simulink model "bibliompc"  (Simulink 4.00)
settings: Solver=ode45  StartTime=0.0  StopTime=10.0  RelTol=1e-3
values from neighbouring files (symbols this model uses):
  m = p    (= 10)    [scr.m]    (also in Smpc.m = mp(1:max(size(mp))-1); demo1dat.m = 4; demo2dat.m = 3; essai1dat.m = 4)
  model = [y(2:ly); 1; 1; .1]    [scr.m]    (also in Smpc.m = modelpd(:,1:nu); essai2dat.m = tfd2step(1.6,delt,1,g); mynlcmpc.m = modelpd(:,1:nu); mynlcmpc2.m = modelpd(:,1:nu))
  p = 10    [scr.m]    (also in Smpc.m = mp(max(size(mp))); demo1dat.m; demo2dat.m; essai1dat.m)
  ulim = [-4 4 .5]    [scr.m]    (also in Smpc.m = [-inf*ones(1,nu) inf*ones(1,nu) 1e6*ones(1,nu)]; essai2dat.m = [-5 40 3]; mynlcmpc.m = [-inf*ones(1,nu) inf*ones(1,nu) 1e6*ones(1,nu)]; mynlcmpc2.m = [-inf*ones(1,nu) inf*ones(1,nu) 1e6*ones(1,nu)])
  uwt = 1    [scr.m]    (also in Smpc.m = yuwt(:,ny+1:ny+nu); demo1dat.m = [0 0]; demo2dat.m = 0.6*[1 1]; essai1dat.m = [0 0])
  ylim = [-inf inf]    [scr.m]    (also in Smpc.m = [ylim; ylim(N,:)]; essai2dat.m = [-40 40]; mynlcmpc.m = [ylim; ylim(N,:)]; mynlcmpc2.m = [ylim; ylim(N,:)])
  ywt = 5    [scr.m]    (also in Smpc.m = yuwt(:,1:ny); demo1dat.m = [1 1]; demo2dat.m = [0.2,0,1]; essai1dat.m = [1 1])

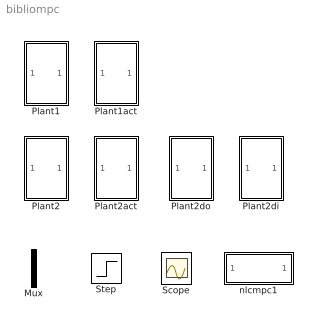
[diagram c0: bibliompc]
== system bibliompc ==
  Mux : Mux  Inputs=2
  Plant1 : Subsystem
  Plant1act : Subsystem
  Plant2 : Subsystem
  Plant2act : Subsystem
  Plant2di : Subsystem
  Plant2do : Subsystem
  Scope : Scope
  Step : Step  Time=0  Before=0  After=1  SampleTime=0
  nlcmpc1 : Subsystem  AncestorBlock=nlmpclib/nlcmpc  mask(Smpc){modelpd=[model []], yuwt=[ywt uwt], mp=[m p], yulim=[ylim ulim], tfilter=[], ud0=[0 []]}
      mask help: Masked MATLAB function block calls nlcmpc, links CMPC and SIMULINK.

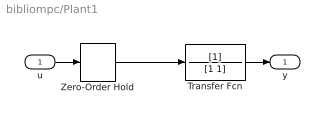
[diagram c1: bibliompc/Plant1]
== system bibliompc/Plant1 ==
  u : Inport  Port=1  LatchInput=off
  Transfer Fcn : TransferFcn  Numerator=[1]  Denominator=[1 1]  AbsoluteTolerance=auto  Realization=auto
  Zero-Order Hold : ZeroOrderHold  SampleTime=0.1
  y : Outport  Port=1
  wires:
  Zero-Order Hold/1 -> Transfer Fcn/1
  u/1 -> Zero-Order Hold/1
  Transfer Fcn/1 -> y/1

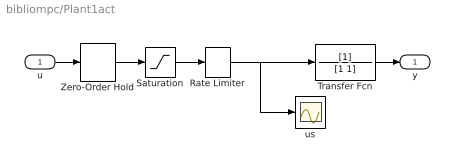
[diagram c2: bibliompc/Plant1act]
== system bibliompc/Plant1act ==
  u : Inport  Port=1  LatchInput=off
  Rate Limiter : RateLimiter  RisingSlewLimit=10  FallingSlewLimit=-10
  Saturation : Saturate  UpperLimit=2  LowerLimit=-2  LinearizeAsGain=on
  Transfer Fcn : TransferFcn  Numerator=[1]  Denominator=[1 1]  AbsoluteTolerance=auto  Realization=auto
  Zero-Order Hold : ZeroOrderHold  SampleTime=0.1
  us : Scope
  y : Outport  Port=1
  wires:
  u/1 -> Zero-Order Hold/1
  Transfer Fcn/1 -> y/1
  Saturation/1 -> Rate Limiter/1
  Zero-Order Hold/1 -> Saturation/1
  Rate Limiter/1 -> Transfer Fcn/1, us/1

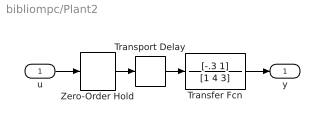
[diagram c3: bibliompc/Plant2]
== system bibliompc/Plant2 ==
  u : Inport  Port=1  LatchInput=off
  Transfer Fcn : TransferFcn  Numerator=[-.3 1]  Denominator=[1 4 3]  AbsoluteTolerance=auto  Realization=auto
  Transport Delay : TransportDelay  DelayTime=.2  InitialInput=0  BufferSize=1024  PadeOrder=0
  Zero-Order Hold : ZeroOrderHold  SampleTime=0.1
  y : Outport  Port=1
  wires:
  Zero-Order Hold/1 -> Transport Delay/1
  Transport Delay/1 -> Transfer Fcn/1
  u/1 -> Zero-Order Hold/1
  Transfer Fcn/1 -> y/1

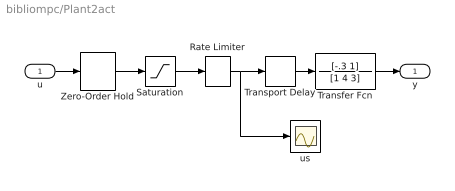
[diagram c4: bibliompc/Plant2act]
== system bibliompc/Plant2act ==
  u : Inport  Port=1  LatchInput=off
  Rate Limiter : RateLimiter  RisingSlewLimit=5  FallingSlewLimit=-5
  Saturation : Saturate  UpperLimit=4  LowerLimit=-4  LinearizeAsGain=on
  Transfer Fcn : TransferFcn  Numerator=[-.3 1]  Denominator=[1 4 3]  AbsoluteTolerance=auto  Realization=auto
  Transport Delay : TransportDelay  DelayTime=.2  InitialInput=0  BufferSize=1024  PadeOrder=0
  Zero-Order Hold : ZeroOrderHold  SampleTime=0.1
  us : Scope
  y : Outport  Port=1
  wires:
  Transport Delay/1 -> Transfer Fcn/1
  u/1 -> Zero-Order Hold/1
  Transfer Fcn/1 -> y/1
  Saturation/1 -> Rate Limiter/1
  Zero-Order Hold/1 -> Saturation/1
  Rate Limiter/1 -> Transport Delay/1, us/1

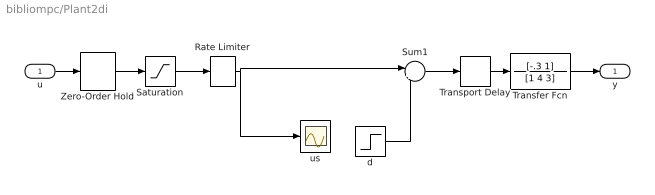
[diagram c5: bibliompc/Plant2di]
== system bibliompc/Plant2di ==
  u : Inport  Port=1  LatchInput=off
  Rate Limiter : RateLimiter  RisingSlewLimit=5  FallingSlewLimit=-5
  Saturation : Saturate  UpperLimit=4  LowerLimit=-4  LinearizeAsGain=on
  Sum1 : Sum  Inputs=|++  SaturateOnIntegerOverflow=on
  Transfer Fcn : TransferFcn  Numerator=[-.3 1]  Denominator=[1 4 3]  AbsoluteTolerance=auto  Realization=auto
  Transport Delay : TransportDelay  DelayTime=.2  InitialInput=0  BufferSize=1024  PadeOrder=0
  Zero-Order Hold : ZeroOrderHold  SampleTime=0.1
  d : Step  Time=4  Before=0  After=1  SampleTime=0
  us : Scope
  y : Outport  Port=1
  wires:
  u/1 -> Zero-Order Hold/1
  Saturation/1 -> Rate Limiter/1
  Zero-Order Hold/1 -> Saturation/1
  Rate Limiter/1 -> us/1, Sum1/1
  d/1 -> Sum1/2
  Transport Delay/1 -> Transfer Fcn/1
  Sum1/1 -> Transport Delay/1
  Transfer Fcn/1 -> y/1

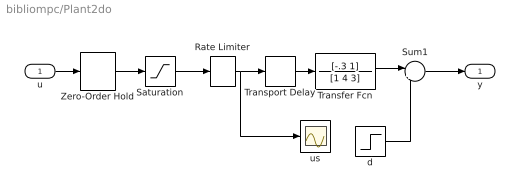
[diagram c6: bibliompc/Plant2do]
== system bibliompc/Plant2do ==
  u : Inport  Port=1  LatchInput=off
  Rate Limiter : RateLimiter  RisingSlewLimit=5  FallingSlewLimit=-5
  Saturation : Saturate  UpperLimit=4  LowerLimit=-4  LinearizeAsGain=on
  Sum1 : Sum  Inputs=|++  SaturateOnIntegerOverflow=on
  Transfer Fcn : TransferFcn  Numerator=[-.3 1]  Denominator=[1 4 3]  AbsoluteTolerance=auto  Realization=auto
  Transport Delay : TransportDelay  DelayTime=.2  InitialInput=0  BufferSize=1024  PadeOrder=0
  Zero-Order Hold : ZeroOrderHold  SampleTime=0.1
  d : Step  Time=4  Before=0  After=1  SampleTime=0
  us : Scope
  y : Outport  Port=1
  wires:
  Transport Delay/1 -> Transfer Fcn/1
  u/1 -> Zero-Order Hold/1
  Saturation/1 -> Rate Limiter/1
  Zero-Order Hold/1 -> Saturation/1
  Rate Limiter/1 -> Transport Delay/1, us/1
  d/1 -> Sum1/2
  Transfer Fcn/1 -> Sum1/1
  Sum1/1 -> y/1

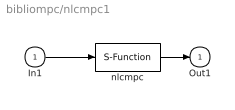
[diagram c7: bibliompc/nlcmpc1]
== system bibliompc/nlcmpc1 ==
  In1 : Inport  Port=1  LatchInput=off
  nlcmpc : S-Function  FunctionName=Smpc  Parameters=modelpd,mp,tfilter,yuwt,ud0,yulim  PortCounts=[]  SFunctionModules=''
  Out1 : Outport  Port=1  InitialOutput=0
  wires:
  In1/1 -> nlcmpc/1
  nlcmpc/1 -> Out1/1
